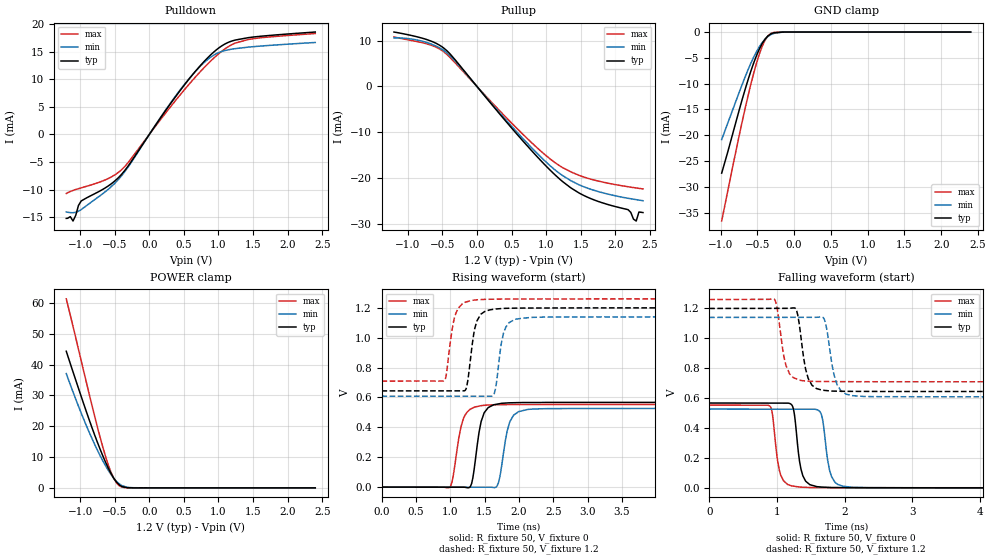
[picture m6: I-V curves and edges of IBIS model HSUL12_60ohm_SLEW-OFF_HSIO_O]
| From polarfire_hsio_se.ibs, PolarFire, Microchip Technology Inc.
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|   Model HSUL12_60ohm_SLEW-OFF_HSIO_O
[Model]   HSUL12_60ohm_SLEW-OFF_HSIO_O
Model_type   Output
Polarity   Non-Inverting
Enable   Active-High
Vmeas =   0.6
Cref =   5p
Rref =   50
Vref =   0.6
|   typ   min   max
C_comp_pullup   1.335e-12   1.335e-12   1.380e-12
C_comp_pulldown  1.335e-12   1.335e-12   1.380e-12
[Temperature Range]  25C   100C   -40C
[Voltage Range]  1.2   1.14   1.26
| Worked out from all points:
|   slope of the pulldown table from 0 to 0.18 V, typ, clamps not added: 54.1 ohm
|   slope of the pullup table from 0 to 0.18 V, typ, clamps not added: 54.3 ohm
|   GND clamp passes 1 mA (typ) near -0.37 V on its own axis
|   POWER clamp passes 1 mA (typ) near -0.44 V on its own axis
|   rising waveform, R_fixture 50, V_fixture 0: 20-80 % time 115ps typ, 121ps min, 126ps max; typ from 0 V to 0.567 V
|   rising waveform, R_fixture 50, V_fixture 1.2: 20-80 % time 106ps typ, 100ps min, 111ps max; typ from 0.644 V to 1.2 V
|   falling waveform, R_fixture 50, V_fixture 0: 20-80 % time 94.1ps typ, 98.8ps min, 93.3ps max; typ from 0.567 V to 0 V
|   falling waveform, R_fixture 50, V_fixture 1.2: 20-80 % time 116ps typ, 125ps min, 113ps max; typ from 1.2 V to 0.644 V
[GND Clamp]
| Voltage   I(typ)   I(min)   I(max)
-984.4mV  -27.36mA   -20.85mA   -36.63mA
-708.7mV  -13.22mA   -10.27mA   -17.58mA
-630mV    -9.442mA   -7.443mA   -12.61mA
-551.3mV  -6.071mA   -4.927mA   -8.091mA
-472.5mV  -3.303mA   -2.86mA    -4.278mA
-433.1mV  -2.213mA   -2.035mA   -2.745mA
-393.7mV  -1.354mA   -1.365mA   -1.538mA
-354.4mV  -738.1uA   -853.7uA   -711.7uA
-315mV    -352.4uA   -492.8uA   -262uA
-157.5mV  -6.952uA   -25.53uA   -1.531uA
-39.38mV  -223.3nA   -1.393uA   -60.97nA
2.4V      0A         0A         0A
[POWER Clamp]
| Voltage   I(typ)   I(min)   I(max)
-1.2V     44.33mA    37.08mA    61.33mA
-1.063V   34.96mA    28.78mA    48.72mA
-905.6mV  24.47mA    19.99mA    33.89mA
-787.5mV  17.03mA    14mA       23.06mA
-669.4mV  10.26mA    8.667mA    13.03mA
-590.6mV  6.299mA    5.605mA    7.313mA
-551.3mV  4.569mA    4.255mA    4.935mA
-472.5mV  1.839mA    2.031mA    1.558mA
-433.1mV  941.2uA    1.284mA    654.9uA
-315mV    34.81uA    149.8uA    11.13uA
-236.2mV  2.462uA    44.69uA    773.7nA
2.4V      0A         0A         0A
[Pullup]
| Voltage   I(typ)   I(min)   I(max)
-1.2V     11.9mA     10.61mA    10.83mA
-748.1mV  10.36mA    9.712mA    9.406mA
-433.1mV  7.788mA    7.317mA    6.984mA
675mV     -12.08mA   -11.54mA   -10.61mA
1.239V    -20.78mA   -19.46mA   -17.73mA
1.633V    -24.41mA   -22.39mA   -20.18mA
2.184V    -26.9mA    -24.42mA   -21.9mA
2.224V    -27.5mA    -24.52mA   -21.99mA
2.263V    -28.97mA   -24.62mA   -22.08mA
2.303V    -29.38mA   -24.71mA   -22.17mA
2.342V    -27.42mA   -24.81mA   -22.25mA
2.4V      -27.54mA   -24.95mA   -22.37mA
[Pulldown]
| Voltage   I(typ)   I(min)   I(max)
-1.2V     -15.23mA   -14.05mA   -10.71mA
-1.142V   -14.92mA   -14.19mA   -10.35mA
-1.103V   -15.71mA   -14.2mA    -10.16mA
-984.4mV  -12.07mA   -13.64mA   -9.691mA
-590.6mV  -9.322mA   -9.923mA   -7.979mA
-393.7mV  -7.136mA   -7.387mA   -6.321mA
412.5mV   7.41mA     7.535mA    6.671mA
675mV     11.59mA    11.57mA    10.54mA
900mV     14.6mA     14.14mA    13.48mA
1.125V    16.63mA    15.34mA    15.81mA
1.436V    17.59mA    15.87mA    17.26mA
2.4V      18.6mA     16.71mA    18.33mA
[Ramp]
dV/dt_r   0.340474/0.114795n  0.316039/0.120797n  0.332062/0.126194n
dV/dt_f   0.333655/0.115787n  0.318831/0.124724n  0.330436/0.1129n
R_load = 50
[Rising Waveform]
R_fixture = 50
V_fixture = 0
V_fixture_min = 0
V_fixture_max = 0
| Time   V(typ)   V(min)   V(max)
0s        1.164uV    1.448uV    1.745uV
993ps     -681uV     -536.6uV   -2.294mV
1.155ns   -792.3uV   -624.4uV   400.7mV
1.272ns   -4.309mV   -687.8uV   513.2mV
1.329ns   59.73mV    -718.7uV   529.6mV
1.459ns   450.2mV    -789.2uV   545.8mV
1.683ns   555.4mV    7.745mV    551.3mV
1.868ns   564.2mV    437.4mV    552.2mV
2.132ns   566.2mV    520.2mV    552.7mV
10ns      567.5mV    526.7mV    553.4mV
[Rising Waveform]
R_fixture = 50
V_fixture = 1.2
V_fixture_min = 1.14
V_fixture_max = 1.26
| Time   V(typ)   V(min)   V(max)
0s        643.9mV    608.6mV    709.3mV
914ps     644.2mV    608.6mV    712.2mV
1.06ns    644.3mV    608.6mV    1.13V
1.213ns   646.1mV    608.5mV    1.236V
1.259ns   719.9mV    608.5mV    1.243V
1.383ns   1.103V     608.5mV    1.254V
1.628ns   1.19V      614.5mV    1.258V
1.777ns   1.196V     1.032V     1.259V
2.023ns   1.198V     1.129V     1.259V
10ns      1.2V       1.14V      1.26V
[Falling Waveform]
R_fixture = 50
V_fixture = 0
V_fixture_min = 0
V_fixture_max = 0
| Time   V(typ)   V(min)   V(max)
0s        567.5mV    526.7mV    553.4mV
895ps     566.9mV    526.3mV    547mV
1.036ns   566.8mV    526.3mV    118.1mV
1.228ns   548.9mV    526.2mV    12.48mV
1.338ns   169.4mV    526.1mV    5.008mV
1.425ns   44.6mV     526.1mV    3.404mV
1.644ns   5.887mV    504mV      1.547mV
1.781ns   2.809mV    113mV      961.1uV
1.973ns   1.477mV    11.28mV    885.9uV
10ns      1.935uV    3.313uV    3.463uV
[Falling Waveform]
R_fixture = 50
V_fixture = 1.2
V_fixture_min = 1.14
V_fixture_max = 1.26
| Time   V(typ)   V(min)   V(max)
0s        1.2V       1.14V      1.26V
957ps     1.201V     1.14V      1.264V
1.134ns   1.201V     1.141V     819mV
1.278ns   1.198V     1.141V     731.1mV
1.357ns   1.003V     1.141V     717.9mV
1.519ns   686.1mV    1.141V     712.7mV
1.701ns   652.1mV    1.127V     711.2mV
1.889ns   646.6mV    690.8mV    710.7mV
2.112ns   645.4mV    617mV      710.3mV
10ns      643.9mV    608.6mV    709.3mV
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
